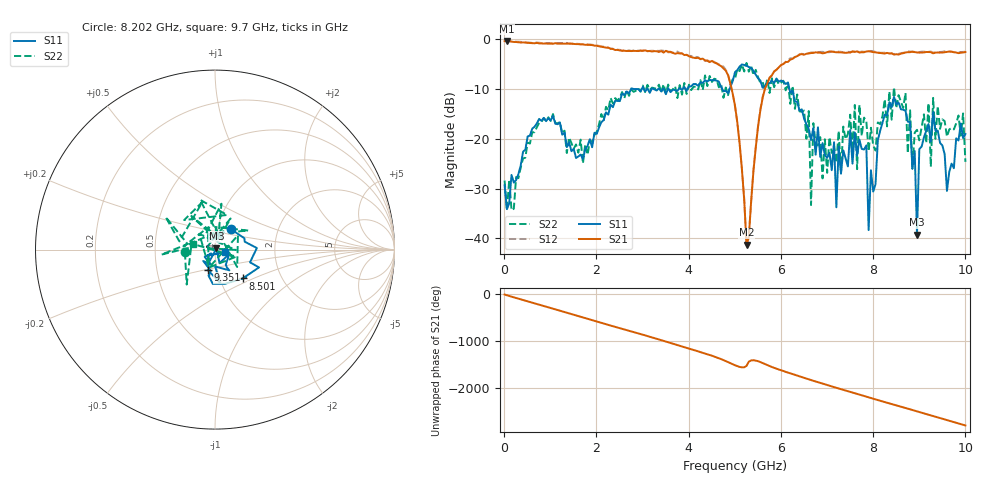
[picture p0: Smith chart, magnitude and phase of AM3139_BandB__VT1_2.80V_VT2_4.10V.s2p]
! Date/Time: Tue, Nov 13, 2018 5:00 PM
! Network Analyzer: Agilent Technologies E8364B Rev: A.07.50.67
! Sweep from 0.010 to 10.000 GHz, 201 Points, Sweep Type: LIN
! Power Supply: 2.801 V, 0.000 A
# Hz S DB R 50
!freq MagS11 AngS11 MagS21 AngS21 MagS12 AngS12 MagS22 AngS22
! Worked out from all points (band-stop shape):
!   201 points, 10 MHz to 10 GHz, reference 50 ohm
!   highest |S21| = -0.34 dB at 59.95 MHz (marker M1); lowest = -41.3 dB at 5.255 GHz (marker M2)
!   |S21| within 3 dB of the highest: start of sweep to 3.998 GHz; 6.357 GHz to end of sweep
!   lowest |S11| = -39.2 dB at 8.951 GHz (marker M3), VSWR 1.02, Z = 50.8 + j0.743 ohm
!   |S11| at or under -10 dB: start of sweep to 2.75 GHz; 3.569 GHz to 3.785 GHz (215.9 MHz wide, 5.87 % of centre); 6.185 GHz to end of sweep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
!   |S22| runs from -34.4 to -4.7 dB; largest |S21 - S12| = 0.032
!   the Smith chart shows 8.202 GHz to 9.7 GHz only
!   S11 on the Smith chart (normalised r, x): 8.202 GHz: 1.16, +0.27; 8.501 GHz: 1.28, -0.43; 9.351 GHz: 0.90, -0.21; 9.7 GHz: 1.12, -0.03
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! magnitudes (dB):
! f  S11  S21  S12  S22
! 10 MHz  -29.3  -0.4  -0.2  -28.4
! 59.95 MHz  -34.1  -0.3  -0.2  -34.4
! 859.2 MHz  -15.8  -0.8  -0.7  -15.8
! 1.708 GHz  -24.0  -1.0  -0.9  -24.9
! 3.357 GHz  -9.8  -2.5  -2.3  -9.1
! 5.005 GHz  -6.6  -13.3  -13.5  -7.9
! 5.255 GHz  -5.3  -41.3  -41.6  -4.7
! 5.654 GHz  -9.4  -9.9  -9.7  -10.1
! 6.603 GHz  -18.0  -2.8  -2.8  -14.4
! 6.653 GHz  -20.2  -2.7  -2.6  -33.3
! 6.703 GHz  -17.8  -2.7  -2.6  -16.8
! 7.203 GHz  -33.8  -2.6  -2.4  -24.8
! 7.852 GHz  -21.3  -2.4  -2.4  -16.4
! 7.902 GHz  -38.3  -2.4  -2.4  -22.5
! 8.202 GHz  -16.8  -2.8  -2.7  -15.5
! 8.352 GHz  -12.6  -2.8  -2.8  -10.5
! 8.501 GHz  -13.1  -3.0  -2.8  -13.8
! 8.951 GHz  -39.2  -2.6  -2.5  -18.2
! 9.001 GHz  -22.0  -2.7  -2.5  -20.3
! 9.351 GHz  -18.4  -2.7  -2.6  -20.0
! 9.7 GHz  -25.0  -2.5  -2.5  -17.8
! 10 GHz  -19.0  -2.5  -2.5  -24.6
